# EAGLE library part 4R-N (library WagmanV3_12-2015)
Array Chip Resistor Source: RS Component / Phycomp
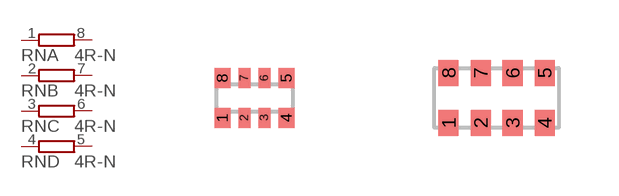
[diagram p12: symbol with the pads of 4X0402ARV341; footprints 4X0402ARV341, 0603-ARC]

Designator prefix RN; gates A=R1NV B=R1NV C=R1NV D=R1NV

## 4R-N0402ARV341  [4X0402ARV341]
1  A:1  pas
2  B:1  pas
3  C:1  pas
4  D:1  pas
5  D:2  pas
6  C:2  pas
7  B:2  pas
8  A:2  pas

## 4R-N0603-ARC  [0603-ARC]
Pads as for 4X0402ARV341

## 4R-N0603-ARV  [0603-ARV]
Pads as for 4X0402ARV341

## 4R-NCAT16  [CAT16]
Pads as for 4X0402ARV341

## 4R-NCAY16  [CAY16]
Pads as for 4X0402ARV341

## 4R-NEXB18V  [EXB18V]
Pads as for 4X0402ARV341

## 4R-NEXB28V  [EXB28V]
Pads as for 4X0402ARV341

## 4R-NEXB38V  [EXB38V]
Pads as for 4X0402ARV341

## 4R-NEXBN8V  [EXBN8V]
Pads as for 4X0402ARV341

## 4R-NEXBS8V  [EXBS8V]
Pads as for 4X0402ARV341

## 4R-NEXBV8V  [EXBV8V]
Pads as for 4X0402ARV341

## 4R-NYC124  [YC124]
Pads as for 4X0402ARV341

## Footprint 4X0402ARV341 (pad centres in mm)
Array chip resistor size 4 × 0402 Source: http://docs-europe.electrocomponents.com/webdocs/0114/0900766b80114d99.pdf
smd 0.4 x 0.5: 1 -0.8,-0.5; 4 0.8,-0.5; 5 0.8,0.5; 8 -0.8,0.5
smd 0.3 x 0.5: 2 -0.25,-0.5; 3 0.25,-0.5; 6 0.25,0.5; 7 -0.25,0.5

## Footprint 0603-ARC (pad centres in mm)
Chip Resistor Array size 4 × 0603 concave termination - Phycomp Components Source: RS Components
smd 0.5 x 0.65: 1 -1.2,-0.625; 2 -0.4,-0.625; 3 0.4,-0.625; 4 1.2,-0.625; 5 1.2,0.625; 6 0.4,0.625; 7 -0.4,0.625; 8 -1.2,0.625

## Footprint 0603-ARV (pad centres in mm)
Chip Resistor Array size 4 × 0603 convex termination - Phycomp Components Source: RS Components
smd 0.5 x 0.65: 1 -1.2,-0.625; 2 -0.4,-0.625; 3 0.4,-0.625; 4 1.2,-0.625; 5 1.2,0.625; 6 0.4,0.625; 7 -0.4,0.625; 8 -1.2,0.625

## Footprint CAT16 (pad centres in mm)
BOURNS Chip Resistor Array Source: RS Component / BUORNS
smd 0.5 x 0.65: 1 -1.2,-0.675; 2 -0.4,-0.675; 3 0.4,-0.675; 4 1.2,-0.675; 5 1.2,0.675; 6 0.4,0.675; 7 -0.4,0.675; 8 -1.2,0.675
